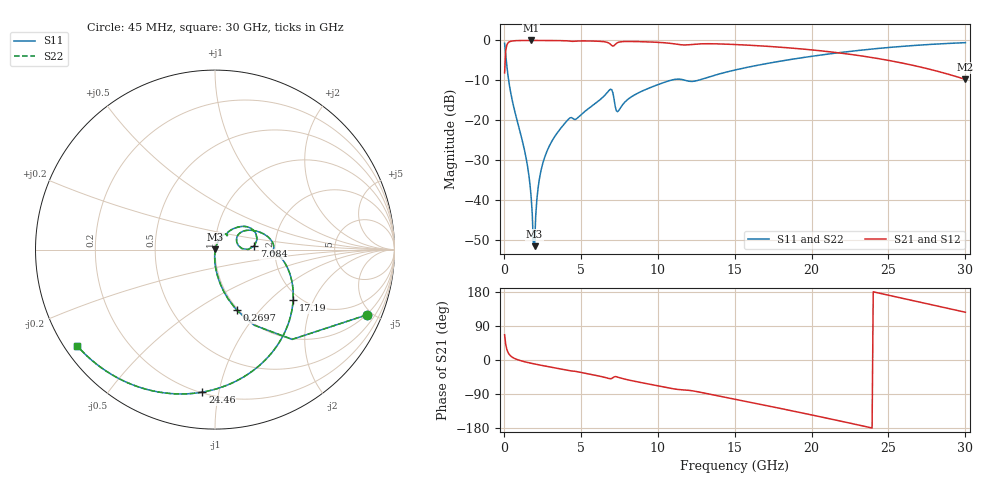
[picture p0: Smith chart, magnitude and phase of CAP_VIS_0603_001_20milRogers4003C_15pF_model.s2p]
! S-parameter model data by Modelithics Inc.  support@modelithics.com  813-866-6335  Tampa FL USA
! S-Parameter data specifications:
! Substrate: 20-mil Rogers 4003C, substrate thickness, H=0.508mm, Dielectric constant, Er=3.75
! PCB Mounting Pad Footprint: Pad width, PadW=0.90mm , Pad length, PadL=1.00mm , Pad gap, PadG (edge-to-edge)=1.00mm , Reference planes=3.0mm apart
! Created Wed Nov 18 13:26:45 2015
# hz S ma R 50
! 2 Port Network Data from SP1.SP block
! freq  magS11  angS11  magS21  angS21  magS12  angS12  magS22  angS22
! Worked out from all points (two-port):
!   401 points, 45 MHz to 30 GHz, reference 50 ohm
!   highest |S21| = -0.02 dB at 1.767 GHz (marker M1); lowest = -9.8 dB at 30 GHz (marker M2)
!   |S21| within 3 dB of the highest: 112.8 MHz to 21.54 GHz (21.43 GHz wide, 198 % of centre)
!   lowest |S11| = -51.5 dB at 1.992 GHz (marker M3), VSWR 1.01, Z = 50.2 + j0.17 ohm
!   |S11| at or under -10 dB: 310.4 MHz to 10.83 GHz (10.52 GHz wide, 189 % of centre); 11.79 GHz to 12.62 GHz (836.7 MHz wide, 6.86 % of centre)
!   |S22| runs from -51.5 to -0.6 dB; largest |S21 - S12| = 0
!   S11 on the Smith chart (normalised r, x): 45 MHz: 0.98, -4.65; 269.7 MHz: 0.98, -0.76; 7.084 GHz: 1.56, +0.07; 17.19 GHz: 1.84, -1.41; 24.46 GHz: 0.21, -0.89; 30 GHz: 0.04, -0.31
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4.5e7  0.9199 -23.3  0.3921 66.7  0.3921 66.7  0.9199 -23.3
2.696625e8  0.3586 -70.3  0.9329 19.6  0.9329 19.6  0.3586 -70.3
5.692125e8  0.1675 -83.0  0.9849 6.7  0.9849 6.7  0.1675 -83.0
1.467862e9  0.03168 -93.2  0.9979 -5.8  0.9979 -5.8  0.03168 -93.2
1.767412e9  0.01119 -90.3  0.9982 -8.6  0.9982 -8.6  0.01119 -90.3
1.8423e9  0.006732 -85.1  0.9982 -9.2  0.9982 -9.2  0.006732 -85.1
1.992075e9  0.002659 39.6  0.9981 -10.5  0.9981 -10.5  0.002659 39.6
2.366512e9  0.02132 71.4  0.9977 -13.5  0.9977 -13.5  0.02132 71.4
2.815838e9  0.04179 70.0  0.9968 -17.0  0.9968 -17.0  0.04179 70.0
4.088925e9  0.09807 59.1  0.988 -26.9  0.988 -26.9  0.09807 59.1
5.062462e9  0.1198 53.3  0.9851 -33.2  0.9851 -33.2  0.1198 53.3
6.859762e9  0.2393 27.3  0.9157 -49.1  0.9157 -49.1  0.2393 27.3
7.084425e9  0.2207 5.4  0.8488 -46.8  0.8488 -46.8  0.2207 5.4
7.458862e9  0.1322 25.0  0.9484 -45.9  0.9484 -45.9  0.1322 25.0
1.007992e10  0.2827 18.3  0.9438 -68.8  0.9438 -68.8  0.2827 18.3
1.50225e10  0.426 -15.7  0.8879 -103.7  0.8879 -103.7  0.426 -15.7
1.719424e10  0.5176 -32.7  0.8416 -121.4  0.8416 -121.4  0.5176 -32.7
2.003996e10  0.6335 -56.3  0.7596 -145.3  0.7596 -145.3  0.6335 -56.3
2.445832e10  0.7973 -95.1  0.5865 175.9  0.5865 175.9  0.7973 -95.1
2.505742e10  0.8167 -100.5  0.5594 170.5  0.5594 170.5  0.8167 -100.5
2.745382e10  0.8843 -122.2  0.4461 148.8  0.4461 148.8  0.8843 -122.2
3e10  0.9364 -145.0  0.3249 126.0  0.3249 126.0  0.9364 -145.0
